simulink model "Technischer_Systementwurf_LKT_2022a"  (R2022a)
settings: Solver=VariableStepAuto  StartTime=0.0  StopTime=10.0  RelTol=1e-3
model workspace (MAT data in the model file):
  PAR_LKT_Temperatur_f64 : Simulink.Parameter (value not decoded)
symbols that are objects in the model workspace (value not decoded): PAR_LKT_Temperatur_f64
undefined symbols (not defined in the file or in its folder): PAR_LKT_Deckenhoehe_f64, PAR_LKT_Etagen_f64, PAR_LKT_Fensterflaeche_f64, PAR_LKT_Grundflaeche_f64, PAR_LKT_Strompreis_f64, PAR_LKT_Temperatur

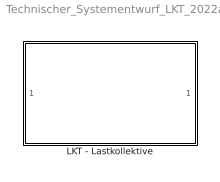
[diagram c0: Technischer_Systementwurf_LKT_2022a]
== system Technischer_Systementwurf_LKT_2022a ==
  LKT - Lastkollektive : Subsystem

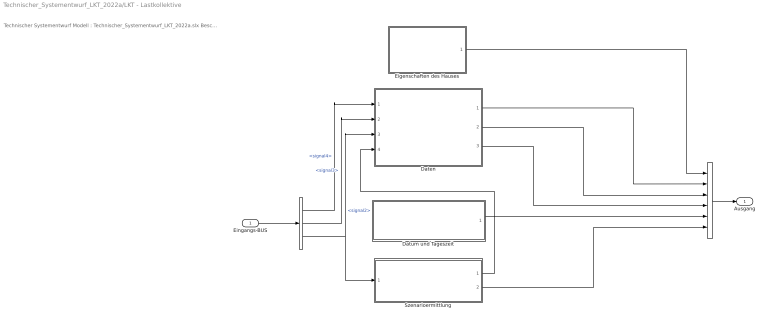
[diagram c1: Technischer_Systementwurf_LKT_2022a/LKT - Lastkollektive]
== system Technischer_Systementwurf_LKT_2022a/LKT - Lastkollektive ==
  note: Technischer Systementwurf Modell : Technischer_Systementwurf_LKT_2022a.slx Beschreibung : Technischer Systementwurf für die Lastkollektive im SoSe 2023 SDE im Simulationsprojekt Einfamilienhaus Implementierung : Simulink (R2022a) Toolbox : Autor : Schartner, David & Stute, Marvin Bemerkung :
  Eingangs-BUS : Inport
  " " : BusSelector  OutputSignals=signal4,signal3,signal2
  "  " : BusCreator  Inputs=6
  Daten : Subsystem
  Datum und Tageszeit : Subsystem
  Eigenschaften des Hauses : Subsystem
  Szenarioermittlung : Subsystem
  Ausgang : Outport
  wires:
  Eigenschaften des Hauses/1(LKT_Eigenschaften_des_Hauses) -> "  "/1
  Daten/1(LKT_Wetterdaten) -> "  "/2
  "  "/1 -> Ausgang/1
  Eingangs-BUS/1 -> " "/1
  " "/2 -> Daten/2(SP_Stromverbrauch)  "<signal3>"
  " "/3 -> Szenarioermittlung/1(LKT_aktuellesDatum), Daten/3(LKT_aktuellesDatum)  "<signal2>"
  Szenarioermittlung/2(LKT_aktuellerStatus) -> "  "/6
  " "/1 -> Daten/1(EEG_Energierzeugung)  "<signal4>"
  Daten/2(LKT_Stromkosten) -> "  "/3
  Daten/3(LKT_Wasserverbrauch) -> "  "/4
  Datum und Tageszeit/1(LKT_aktuellesDatum) -> "  "/5
  Szenarioermittlung/1(Out1) -> Daten/4(LKT_aktuellerStatus)

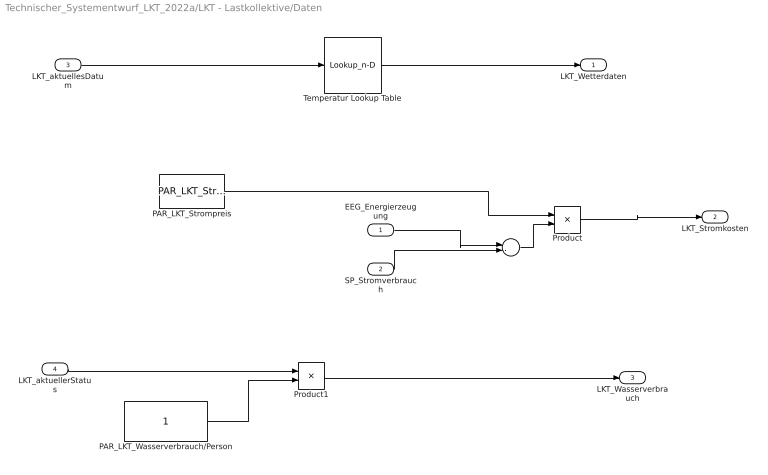
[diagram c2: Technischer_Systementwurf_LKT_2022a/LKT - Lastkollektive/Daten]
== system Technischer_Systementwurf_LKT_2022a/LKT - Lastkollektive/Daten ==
  EEG_Energierzeugung : Inport
  SP_Stromverbrauch : Inport  Port=2
  LKT_aktuellesDatum : Inport  Port=3
  LKT_aktuellerStatus : Inport  Port=4
  " " : Sum  Inputs=|-+
  PAR_LKT_Strompreis : Constant  Value=PAR_LKT_Strompreis_f64
  PAR_LKT_Wasserverbrauch/Person : Constant
  Product : Product
  Product1 : Product
  Temperatur Lookup Table : Lookup_n-D  NumberOfTableDimensions=1  BreakpointsForDimension1=[-5:5]  Table=PAR_LKT_Temperatur  InternalRulePriority=Speed  RndMeth=Simplest
  LKT_Wetterdaten : Outport
  LKT_Stromkosten : Outport  Port=2
  LKT_Wasserverbrauch : Outport  Port=3
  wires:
  PAR_LKT_Strompreis/1 -> Product/1
  LKT_aktuellesDatum/1 -> Temperatur Lookup Table/1
  SP_Stromverbrauch/1 -> " "/2
  Product/1 -> LKT_Stromkosten/1
  EEG_Energierzeugung/1 -> " "/1
  " "/1 -> Product/2
  Product1/1 -> LKT_Wasserverbrauch/1
  Temperatur Lookup Table/1 -> LKT_Wetterdaten/1
  LKT_aktuellerStatus/1 -> Product1/1
  PAR_LKT_Wasserverbrauch/Person/1 -> Product1/2

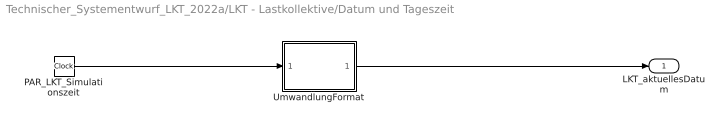
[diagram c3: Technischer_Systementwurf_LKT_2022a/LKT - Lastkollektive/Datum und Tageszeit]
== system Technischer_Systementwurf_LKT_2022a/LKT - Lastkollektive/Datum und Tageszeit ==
  PAR_LKT_Simulationszeit : Clock
  UmwandlungFormat : MATLAB Function  TreatAsAtomicUnit=on
  LKT_aktuellesDatum : Outport
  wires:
  UmwandlungFormat/1(y) -> LKT_aktuellesDatum/1
  PAR_LKT_Simulationszeit/1 -> UmwandlungFormat/1(u)

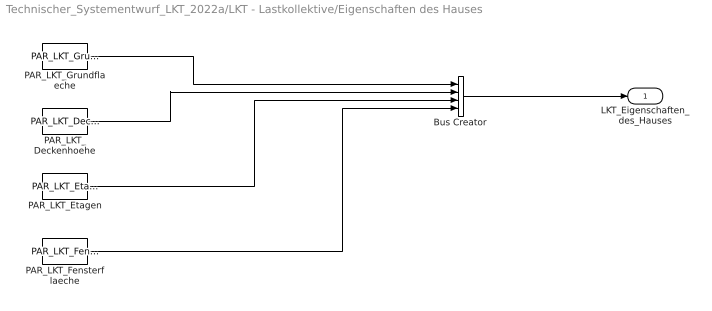
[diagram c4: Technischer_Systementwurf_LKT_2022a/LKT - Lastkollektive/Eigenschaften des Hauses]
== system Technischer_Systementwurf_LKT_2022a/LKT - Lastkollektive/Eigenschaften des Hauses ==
  Bus Creator : BusCreator  Inputs=4
  PAR_LKT_Deckenhoehe : Constant  Value=PAR_LKT_Deckenhoehe_f64
  PAR_LKT_Etagen : Constant  Value=PAR_LKT_Etagen_f64
  PAR_LKT_Fensterflaeche : Constant  Value=PAR_LKT_Fensterflaeche_f64
  PAR_LKT_Grundflaeche : Constant  Value=PAR_LKT_Grundflaeche_f64
  LKT_Eigenschaften_des_Hauses : Outport
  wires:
  PAR_LKT_Grundflaeche/1 -> Bus Creator/1
  PAR_LKT_Deckenhoehe/1 -> Bus Creator/2
  PAR_LKT_Etagen/1 -> Bus Creator/3
  PAR_LKT_Fensterflaeche/1 -> Bus Creator/4
  Bus Creator/1 -> LKT_Eigenschaften_des_Hauses/1

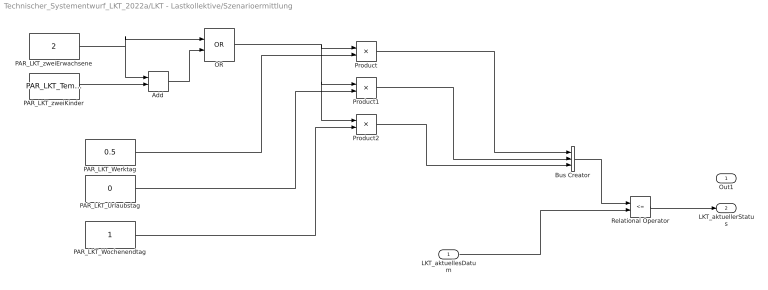
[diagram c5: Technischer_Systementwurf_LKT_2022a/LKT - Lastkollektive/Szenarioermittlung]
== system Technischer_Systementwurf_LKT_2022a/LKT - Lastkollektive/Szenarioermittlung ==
  LKT_aktuellesDatum : Inport
  Add : Sum
  Bus Creator : BusCreator  Inputs=3
  OR : Logic  Operator=OR  AllPortsSameDT=off  OutDataTypeStr=boolean
  PAR_LKT_Urlaubstag : Constant  Value=0
  PAR_LKT_Werktag : Constant  Value=0.5
  PAR_LKT_Wochenendtag : Constant
  PAR_LKT_zweiErwachsene : Constant  Value=2
  PAR_LKT_zweiKinder : Constant  Value=PAR_LKT_Temperatur_f64
  Product : Product
  Product1 : Product
  Product2 : Product
  Relational Operator : RelationalOperator  Operator=<=  OutDataTypeStr=boolean  RndMeth=Simplest
  Out1 : Outport
  LKT_aktuellerStatus : Outport  Port=2
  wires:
  OR/1 -> Product2/1, Product1/1, Product/1
  PAR_LKT_Werktag/1 -> Product/2
  PAR_LKT_Urlaubstag/1 -> Product1/2
  PAR_LKT_Wochenendtag/1 -> Product2/2
  Relational Operator/1 -> LKT_aktuellerStatus/1
  Product/1 -> Bus Creator/1
  LKT_aktuellesDatum/1 -> Relational Operator/2
  PAR_LKT_zweiErwachsene/1 -> OR/1, Add/1
  Bus Creator/1 -> Relational Operator/1
  PAR_LKT_zweiKinder/1 -> Add/2
  Product2/1 -> Bus Creator/3
  Add/1 -> OR/2
  Product1/1 -> Bus Creator/2

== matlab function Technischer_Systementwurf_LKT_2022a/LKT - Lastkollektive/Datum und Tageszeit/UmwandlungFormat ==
function y = fcn(u)

y = u;
